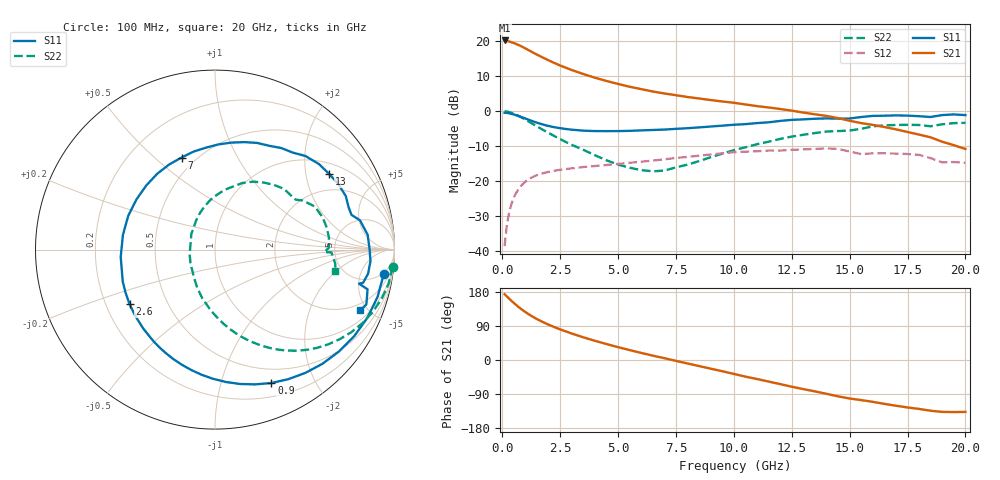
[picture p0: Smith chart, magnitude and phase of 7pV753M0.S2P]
! Infineon Technologies  Discrete & RF Semiconductors
! bfp620
! VCE = 0.75 V,  IC =  3.0 mA
! Common Emitter S-Parameters:  Sep 2002
# GHz  S  MA  R  50
!  f  S11  S21  S12  S22
! GHz  MAG  ANG  MAG  ANG  MAG  ANG  MAG  ANG
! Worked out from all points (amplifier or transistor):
!   59 points, 100 MHz to 20 GHz, reference 50 ohm
!   highest |S21| = 20.1 dB at 100 MHz (marker M1)
!   |S21| within 3 dB of that: start of sweep to 1.202 GHz
!   unconditionally stable (mu >= 1): 5.415 GHz to 12.3 GHz; 14.46 GHz to 15.75 GHz; 16.83 GHz to end of sweep
!   at 1 GHz: K = 0.23, MSG = 19.0 dB, |S12| = -20.1 dB
!   at 5.5 GHz: K = 1.01, MAG = 10.3 dB, |S12| = -14.7 dB
!   at 20 GHz: K = 1.66, MAG = -2.8 dB, |S12| = -14.7 dB
!   S11 on the Smith chart (normalised r, x): 100 MHz: 4, -12; 900 MHz: 0.34, -1.45; 2.6 GHz: 0.30, -0.27; 7 GHz: 0.42, +0.61; 13 GHz: 1.34, +2.71; 20 GHz: 1.52, -4.49
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0.1  0.95 -8.3  10.16 173.4  0.0119 86.4  0.9943 -5.6
0.3  0.9302 -24.0  9.813 161.7  0.0366 76.7  0.9683 -16.4
0.5  0.8942 -39.4  9.324 150.4  0.0586 67.8  0.9174 -26.6
0.7  0.8519 -53.7  8.754 140.0  0.0772 59.9  0.8556 -35.7
0.9  0.8067 -67.1  8.134 130.7  0.0925 52.8  0.7895 -43.9
1.1  0.7618 -79.4  7.504 122.4  0.1048 46.7  0.7237 -51.1
1.3  0.7202 -90.8  6.909 114.8  0.1146 41.4  0.6614 -57.5
1.6  0.6674 -106.1  6.132 104.7  0.1256 34.9  0.5787 -65.7
2  0.6143 -124.1  5.296 93.2  0.1362 28.3  0.4888 -75.1
2.6  0.5647 -147.4  4.329 78.5  0.1473 20.8  0.3837 -87.5
3  0.544 -160.9  3.849 69.8  0.1531 16.6  0.3308 -95.2
3.5  0.5268 -175.6  3.379 59.9  0.1596 12.4  0.2808 -104.5
4  0.5195 171.0  2.993 50.7  0.165 8.6  0.2351 -114.9
5  0.5193 147.3  2.437 33.9  0.1771 2.5  0.1731 -136.7
6  0.5312 127.3  2.057 18.7  0.1902 -3.4  0.1442 -167.3
7  0.5457 109.9  1.784 4.8  0.2056 -9.2  0.142 161.3
8.5  0.5863 88.1  1.513 -16.0  0.2321 -19.9  0.194 122.7
10.5  0.6527 62.3  1.244 -43.9  0.2645 -38.0  0.3053 88.0
13  0.7629 33.6  0.954 -76.9  0.2852 -60.5  0.4605 54.3
13.5  0.7784 28.0  0.9 -82.8  0.2887 -65.5  0.4866 48.0
17  0.8686 -4.2  0.55 -120.7  0.2479 -95.9  0.6347 11.0
20  0.878 -22.7  0.289 -137.0  0.1833 -113.2  0.6804 -10.0
